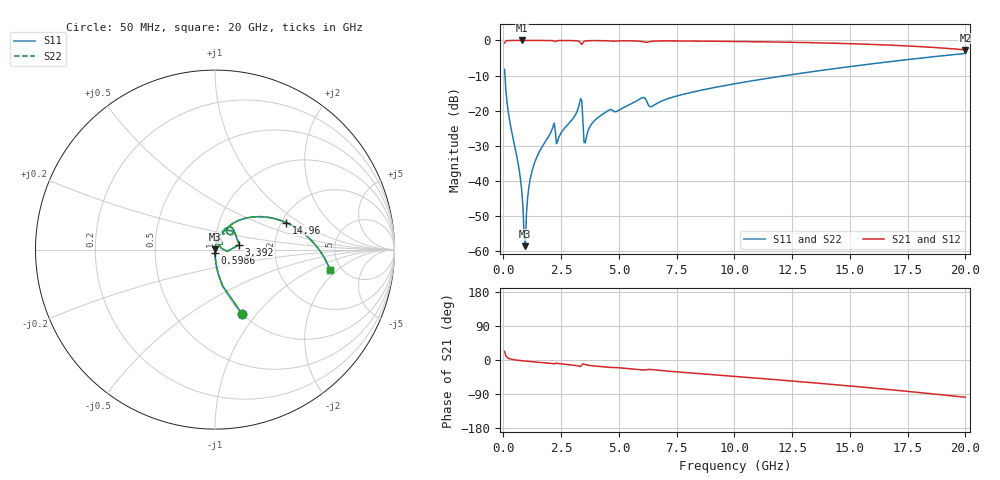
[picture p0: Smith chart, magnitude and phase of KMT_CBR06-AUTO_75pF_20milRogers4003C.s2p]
! Data measured by Modelithics Inc. support@modelithics.com 813-866-6335
! KEMET CBR06-AUTO 75pF, Pad Width= 0.851mm, Pad Length= 0.64mm, Pad Gap= 0.62mm, 20mil Rogers 4003C substrate Data, January 2022
# hz S ma R 50
! 2 Port Network Data from SP1.SP block
! freq  magS11  angS11  magS21  angS21  magS12  angS12  magS22  angS22
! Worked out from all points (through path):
!   401 points, 50 MHz to 20 GHz, reference 50 ohm
!   highest |S21| = 0.00 dB at 798.1 MHz (marker M1); lowest = -2.7 dB at 20 GHz (marker M2)
!   group delay of S21, straight-line fit = 13.6 ps
!   lowest |S11| = -58.6 dB at 947.8 MHz (marker M3), VSWR 1.00, Z = 50.1 + j0.104 ohm
!   |S11| at or under -10 dB: 66.01 MHz to 12.21 GHz (12.14 GHz wide, 198 % of centre)
!   |S22| runs from -58.6 to -3.7 dB; largest |S21 - S12| = 0
!   S11 on the Smith chart (normalised r, x): 50 MHz: 1.00, -0.84; 598.6 MHz: 1.00, -0.04; 3.392 GHz: 1.31, +0.07; 14.96 GHz: 2.11, +0.78; 20 GHz: 4.06, -1.65
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5e7  0.3884 -67.2  0.9211 22.7  0.9211 22.7  0.3884 -67.2
2.495e8  0.0784 -86.0  0.9966 3.8  0.9966 3.8  0.0784 -86.0
5.98625e8  0.02067 -89.5  0.9994 -0.6  0.9994 -0.6  0.02067 -89.5
7.98125e8  0.0069 -88.2  0.9995 -2.0  0.9995 -2.0  0.0069 -88.2
8.48e8  0.004103 -85.7  0.9995 -2.3  0.9995 -2.3  0.004103 -85.7
9.4775e8  0.001179 62.1  0.9995 -2.9  0.9995 -2.9  0.001179 62.1
1.197125e9  0.01217 83.1  0.9993 -4.2  0.9993 -4.2  0.01217 83.1
1.596125e9  0.02765 82.2  0.9988 -6.3  0.9988 -6.3  0.02765 82.2
2.14475e9  0.05934 72.0  0.9897 -9.7  0.9897 -9.7  0.05934 72.0
2.394125e9  0.04126 74.1  0.9944 -9.4  0.9944 -9.4  0.04126 74.1
3.291875e9  0.1261 59.4  0.9621 -16.7  0.9621 -16.7  0.1261 59.4
3.391625e9  0.1378 11.7  0.8733 -13.3  0.8733 -13.3  0.1378 11.7
3.591125e9  0.04223 61.5  0.9877 -12.9  0.9877 -12.9  0.04223 61.5
3.890375e9  0.06937 71.6  0.9939 -15.4  0.9939 -15.4  0.06937 71.6
4.53875e9  0.1006 66.7  0.9874 -19.1  0.9874 -19.1  0.1006 66.7
5.985125e9  0.1517 55.5  0.9668 -26.2  0.9668 -26.2  0.1517 55.5
6.73325e9  0.1317 59.1  0.983 -27.3  0.983 -27.3  0.1317 59.1
1.0025e10  0.242 46.1  0.9673 -43.3  0.9673 -43.3  0.242 46.1
1.336662e10  0.3592 29.5  0.9289 -59.9  0.9289 -59.9  0.3592 29.5
1.496262e10  0.4227 20.9  0.9004 -68.4  0.9004 -68.4  0.4227 20.9
1.670825e10  0.4979 10.9  0.8585 -78.2  0.8585 -78.2  0.4979 10.9
2e10  0.6533 -10.3  0.734 -98.3  0.734 -98.3  0.6533 -10.3
